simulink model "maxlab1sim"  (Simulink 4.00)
settings: Solver=ode45  SolverMode=SingleTasking  StartTime=0.0  StopTime=2  FixedStep=0.001  RelTol=1e-3
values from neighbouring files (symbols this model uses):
  C = lC    [initlab1sim.m]
  dDZ = 0.1    [initlab1sim.m]
  dzpos = 0    [initlab1sim.m]
  DZPOS = 0    [initlab1sim.m]
  GAM = lGAM    [initlab1sim.m]
  h = 0.001    [dfa.m]    (also in initlab1sim.m)
  K = lK    [initlab1sim.m]    (also in lqed.m = Phi*Kf+Kv)
  Lc = lLc    (= 1)    [initlab1sim.m]
  Le = lLe    [initlab1sim.m]
  overlap = 0    [fix_opencfg.m]    (also in fixopencfg.m; initlab1sim.m)
  OVERLAP = 2    [initlab1sim.m]
  PHI = lPHI    [initlab1sim.m]
  tl = -1.3    [initlab1sim.m]
  TL = + 1.3    (= 1.3)    [initlab1sim.m]
  tu = 1.0    (= 1)    [initlab1sim.m]
  TU = - 1.0    (= -1)    [initlab1sim.m]
undefined symbols (not defined in the file or in its folder): SimDen, SimNum
libraries: simulink3 x2, simulink_extras x1

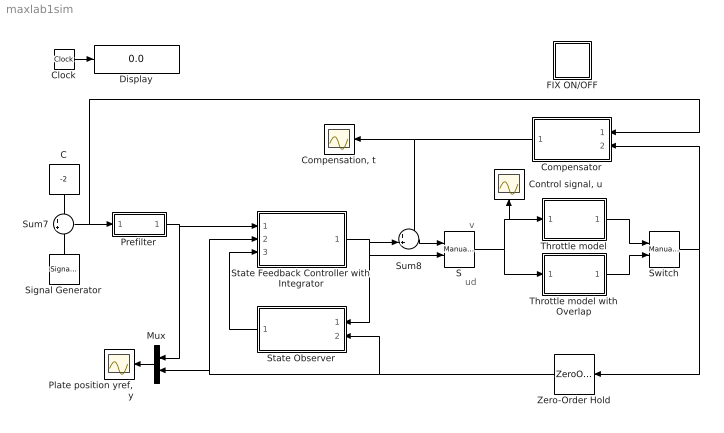
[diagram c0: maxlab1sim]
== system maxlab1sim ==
  note: v
  note: ud
  C : Constant  Orientation=down  Value=-2
  Clock : Clock
  "Compensation, t" : Scope
  Compensator : Subsystem  Orientation=left
  "Control signal, u" : Scope
  Display : Display
  FIX ON/OFF : Subsystem  Description=Fix ON/OFF
  Mux : Mux  Orientation=left  Inputs=2
  "Plate position yref, y" : Scope
  Prefilter : Subsystem
  S : simulink3/Nonlinear/Manual Switch  sw=0  action=0
  Signal Generator : SignalGenerator  Orientation=up  WaveForm=square  Amplitude=2  Frequency=1  Units=Hertz
  State Feedback Controller with Integrator : Subsystem
  State Observer : Subsystem  Orientation=left
  Sum7 : Sum  Inputs=++  SaturateOnIntegerOverflow=on
  Sum8 : Sum  Inputs=++|  SaturateOnIntegerOverflow=on
  Switch : simulink3/Nonlinear/Manual Switch  sw=1  action=0
  Throttle model : Subsystem
  Throttle model with Overlap : Subsystem
  Zero-Order Hold : ZeroOrderHold  Orientation=left  SampleTime=h
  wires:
  Signal Generator/1 -> Sum7/2
  Prefilter/1(rfiltered) -> Mux/1, State Feedback Controller with Integrator/1(yr)
  Mux/1 -> "Plate position yref, y"/1
  Zero-Order Hold/1 -> State Observer/2(y), Mux/2, State Feedback Controller with Integrator/2(y)
  State Observer/1(xhat) -> State Feedback Controller with Integrator/3(xhat)
  Sum7/1 -> Prefilter/1(r), Compensator/1(ref.value)
  Switch/1 -> Zero-Order Hold/1, Compensator/2(y)
  Sum8/1 -> S/1
  State Feedback Controller with Integrator/1(ud) -> Sum8/2, S/2, State Observer/1(u)
  Throttle model with Overlap/1(y) -> Switch/2
  Throttle model/1(y) -> Switch/1
  S/1 -> Throttle model/1(u), "Control signal, u"/1, Throttle model with Overlap/1(u)
  Compensator/1(t) -> Sum8/1, "Compensation, t"/1
  Clock/1 -> Display/1
  C/1 -> Sum7/1

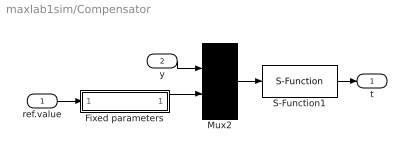
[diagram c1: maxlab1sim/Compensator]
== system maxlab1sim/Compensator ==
  ref.value : Inport  Port=1  LatchInput=off
  y : Inport  Port=2  LatchInput=off
  Fixed parameters : Subsystem
  Mux2 : Mux  Inputs=2
  S-Function1 : S-Function  FunctionName=compensator2  Parameters=h overlap/2 -overlap/2  PortCounts=[]  SFunctionModules=''
  t : Outport  Port=1
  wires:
  ref.value/1 -> Fixed parameters/1(ref value)
  y/1 -> Mux2/1
  Mux2/1 -> S-Function1/1
  S-Function1/1 -> t/1
  Fixed parameters/1(params) -> Mux2/2

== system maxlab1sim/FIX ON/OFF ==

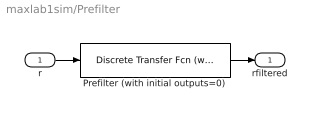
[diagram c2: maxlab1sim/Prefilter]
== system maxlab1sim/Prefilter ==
  r : Inport  Port=1  LatchInput=off
  Prefilter (with initial outputs=0) : simulink_extras/Additional Discrete/Discrete Transfer Fcn (with initial outputs)  N=[21.3 1 -20.3]  D=[835 -1596 763]  U0=[0]  Y0=0  TS=h
  rfiltered : Outport  Port=1
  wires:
  Prefilter (with initial outputs=0)/1 -> rfiltered/1
  r/1 -> Prefilter (with initial outputs=0)/1

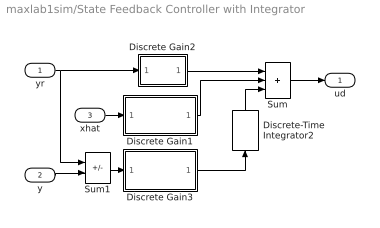
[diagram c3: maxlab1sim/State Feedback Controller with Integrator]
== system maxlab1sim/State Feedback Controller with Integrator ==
  yr : Inport  Port=1  LatchInput=off
  y : Inport  Port=2  LatchInput=off
  xhat : Inport  Port=3  LatchInput=off
  Discrete Gain1 : Subsystem  mask(Discrete Gain){h=h, K=-Le(1:3)}
      mask prompts: h "Sample Time"; K "Gain"
      mask init:
      | s = get_param(gcb,'MaskValueString');
      | s = s(findstr(s,'|')+1:end);
  Discrete Gain2 : Subsystem  mask(Discrete Gain){h=h, K=Lc}
      mask prompts: h "Sample Time"; K "Gain"
      mask init:
      | s = get_param(gcb,'MaskValueString');
      | s = s(findstr(s,'|')+1:end);
  Discrete Gain3 : Subsystem  mask(Discrete Gain){h=h, K=-Le(4)}
      mask prompts: h "Sample Time"; K "Gain"
      mask init:
      | s = get_param(gcb,'MaskValueString');
      | s = s(findstr(s,'|')+1:end);
  Discrete-Time Integrator2 : DiscreteIntegrator  Orientation=up  IntegratorMethod=ForwardEuler  ExternalReset=none  InitialConditionSource=internal  InitialCondition=0  LimitOutput=off  UpperSaturationLimit=inf  LowerSaturationLimit=-inf  ShowSaturationPort=off  ShowStatePort=off  SampleTime=h
  Sum : Sum  Inputs=+++  SaturateOnIntegerOverflow=on
  Sum1 : Sum  Inputs=+-  SaturateOnIntegerOverflow=on
  ud : Outport  Port=1
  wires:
  Discrete Gain1/1(Out1) -> Sum/2
  Discrete-Time Integrator2/1 -> Sum/3
  Sum/1 -> ud/1
  Discrete Gain3/1(Out1) -> Discrete-Time Integrator2/1
  Discrete Gain2/1(Out1) -> Sum/1
  xhat/1 -> Discrete Gain1/1(In1)
  y/1 -> Sum1/2
  yr/1 -> Discrete Gain2/1(In1), Sum1/1
  Sum1/1 -> Discrete Gain3/1(In1)

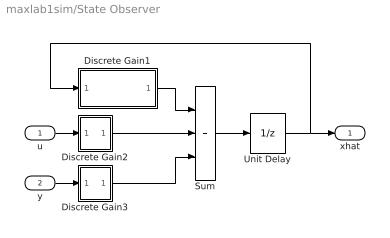
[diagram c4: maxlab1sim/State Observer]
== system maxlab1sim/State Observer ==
  u : Inport  Port=1  LatchInput=off
  y : Inport  Port=2  LatchInput=off
  Discrete Gain1 : Subsystem  mask(Discrete Gain){h=h, K=PHI-K*C}
      mask prompts: h "Sample Time"; K "Gain"
      mask init:
      | s = get_param(gcb,'MaskValueString');
      | s = s(findstr(s,'|')+1:end);
  Discrete Gain2 : Subsystem  mask(Discrete Gain){h=h, K=GAM}
      mask prompts: h "Sample Time"; K "Gain"
      mask init:
      | s = get_param(gcb,'MaskValueString');
      | s = s(findstr(s,'|')+1:end);
  Discrete Gain3 : Subsystem  mask(Discrete Gain){h=h, K=K}
      mask prompts: h "Sample Time"; K "Gain"
      mask init:
      | s = get_param(gcb,'MaskValueString');
      | s = s(findstr(s,'|')+1:end);
  Sum : Sum  Inputs=+++  SaturateOnIntegerOverflow=on
  Unit Delay : UnitDelay  X0=0  SampleTime=h
  xhat : Outport  Port=1
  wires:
  Discrete Gain1/1(Out1) -> Sum/1
  Discrete Gain2/1(Out1) -> Sum/2
  Discrete Gain3/1(Out1) -> Sum/3
  Sum/1 -> Unit Delay/1
  Unit Delay/1 -> Discrete Gain1/1(In1), xhat/1
  u/1 -> Discrete Gain2/1(In1)
  y/1 -> Discrete Gain3/1(In1)

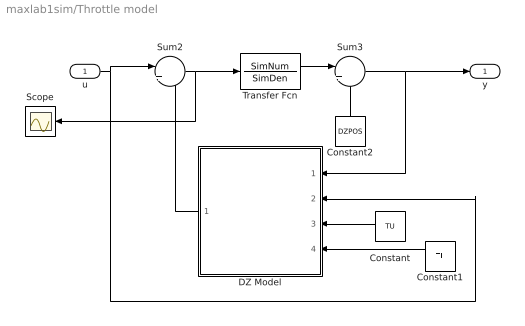
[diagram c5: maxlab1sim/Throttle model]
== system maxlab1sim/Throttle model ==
  u : Inport  Port=1  LatchInput=off
  Constant : Constant  Orientation=left  Value=TU
  Constant1 : Constant  Orientation=left  Value=TL
  Constant2 : Constant  Orientation=up  Value=DZPOS
  DZ Model : Subsystem  Orientation=left
  Scope : Scope
  Sum2 : Sum  Inputs=|++  SaturateOnIntegerOverflow=on
  Sum3 : Sum  Inputs=|++  SaturateOnIntegerOverflow=on
  Transfer Fcn : TransferFcn  Numerator=SimNum  Denominator=SimDen  AbsoluteTolerance=auto  Realization=auto
  y : Outport  Port=1
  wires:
  Sum3/1 -> DZ Model/1(position), y/1
  Constant2/1 -> Sum3/2
  Transfer Fcn/1 -> Sum3/1
  u/1 -> DZ Model/2(torque), Sum2/1
  Constant/1 -> DZ Model/3(TU)
  Constant1/1 -> DZ Model/4(TL)
  Sum2/1 -> Transfer Fcn/1, Scope/1
  DZ Model/1(dz) -> Sum2/2

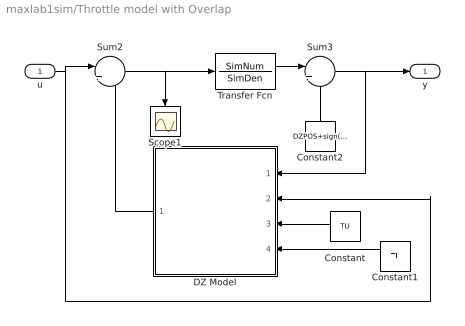
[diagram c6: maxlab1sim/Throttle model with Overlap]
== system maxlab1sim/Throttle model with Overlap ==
  u : Inport  Port=1  LatchInput=off
  Constant : Constant  Orientation=left  Value=TU
  Constant1 : Constant  Orientation=left  Value=TL
  Constant2 : Constant  Orientation=up  Value=DZPOS+sign(TU+TL)*OVERLAP/2
  DZ Model : Subsystem  Orientation=left
  Scope1 : Scope
  Sum2 : Sum  Inputs=|++  SaturateOnIntegerOverflow=on
  Sum3 : Sum  Inputs=|++  SaturateOnIntegerOverflow=on
  Transfer Fcn : TransferFcn  Numerator=SimNum  Denominator=SimDen  AbsoluteTolerance=auto  Realization=auto
  y : Outport  Port=1
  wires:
  Sum3/1 -> DZ Model/1(position), y/1
  Constant2/1 -> Sum3/2
  Transfer Fcn/1 -> Sum3/1
  Sum2/1 -> Scope1/1, Transfer Fcn/1
  Constant1/1 -> DZ Model/4(TL)
  Constant/1 -> DZ Model/3(TU)
  u/1 -> DZ Model/2(torque), Sum2/1
  DZ Model/1(dz) -> Sum2/2

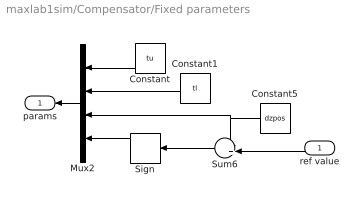
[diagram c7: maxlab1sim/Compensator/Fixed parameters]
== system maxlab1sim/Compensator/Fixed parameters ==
  ref value : Inport  Orientation=left  Port=1  LatchInput=off
  Constant : Constant  Orientation=left  Value=tu
  Constant1 : Constant  Orientation=left  Value=tl
  Constant5 : Constant  Orientation=left  Value=dzpos
  Mux2 : Mux  Orientation=left  Inputs=4
  Sign : Signum  Orientation=left
  Sum6 : Sum  Orientation=left  Inputs=-+|  SaturateOnIntegerOverflow=on
  params : Outport  Orientation=left  Port=1
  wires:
  Sign/1 -> Mux2/4
  Constant/1 -> Mux2/1
  Constant5/1 -> Mux2/3, Sum6/1
  ref value/1 -> Sum6/2
  Sum6/1 -> Sign/1
  Constant1/1 -> Mux2/2
  Mux2/1 -> params/1

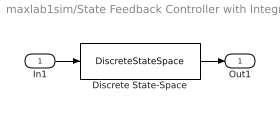
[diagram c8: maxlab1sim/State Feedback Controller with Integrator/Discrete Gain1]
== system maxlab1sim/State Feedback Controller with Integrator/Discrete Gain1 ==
  In1 : Inport  Port=1  LatchInput=off
  Discrete State-Space : DiscreteStateSpace  A=0  B=zeros(1,size(K,2))  C=zeros(size(K,1),1)  D=K  X0=0  SampleTime=h  Realization=auto
  Out1 : Outport  Port=1
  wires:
  Discrete State-Space/1 -> Out1/1
  In1/1 -> Discrete State-Space/1

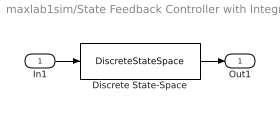
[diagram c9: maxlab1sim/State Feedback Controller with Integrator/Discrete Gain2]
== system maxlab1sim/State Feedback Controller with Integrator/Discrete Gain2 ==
  In1 : Inport  Port=1  LatchInput=off
  Discrete State-Space : DiscreteStateSpace  A=0  B=zeros(1,size(K,2))  C=zeros(size(K,1),1)  D=K  X0=0  SampleTime=h  Realization=auto
  Out1 : Outport  Port=1
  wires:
  Discrete State-Space/1 -> Out1/1
  In1/1 -> Discrete State-Space/1

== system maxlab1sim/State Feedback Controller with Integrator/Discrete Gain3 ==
  In1 : Inport  Port=1  LatchInput=off
  Discrete State-Space : DiscreteStateSpace  A=0  B=zeros(1,size(K,2))  C=zeros(size(K,1),1)  D=K  X0=0  SampleTime=h  Realization=auto
  Out1 : Outport  Port=1
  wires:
  In1/1 -> Discrete State-Space/1
  Discrete State-Space/1 -> Out1/1

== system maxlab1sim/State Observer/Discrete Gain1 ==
  In1 : Inport  Port=1  LatchInput=off
  Discrete State-Space : DiscreteStateSpace  A=0  B=zeros(1,size(K,2))  C=zeros(size(K,1),1)  D=K  X0=0  SampleTime=h  Realization=auto
  Out1 : Outport  Port=1
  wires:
  Discrete State-Space/1 -> Out1/1
  In1/1 -> Discrete State-Space/1

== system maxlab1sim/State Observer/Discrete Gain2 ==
  In1 : Inport  Port=1  LatchInput=off
  Discrete State-Space : DiscreteStateSpace  A=0  B=zeros(1,size(K,2))  C=zeros(size(K,1),1)  D=K  X0=0  SampleTime=h  Realization=auto
  Out1 : Outport  Port=1
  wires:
  In1/1 -> Discrete State-Space/1
  Discrete State-Space/1 -> Out1/1

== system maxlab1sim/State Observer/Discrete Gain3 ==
  In1 : Inport  Port=1  LatchInput=off
  Discrete State-Space : DiscreteStateSpace  A=0  B=zeros(1,size(K,2))  C=zeros(size(K,1),1)  D=K  X0=0  SampleTime=h  Realization=auto
  Out1 : Outport  Port=1
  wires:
  Discrete State-Space/1 -> Out1/1
  In1/1 -> Discrete State-Space/1

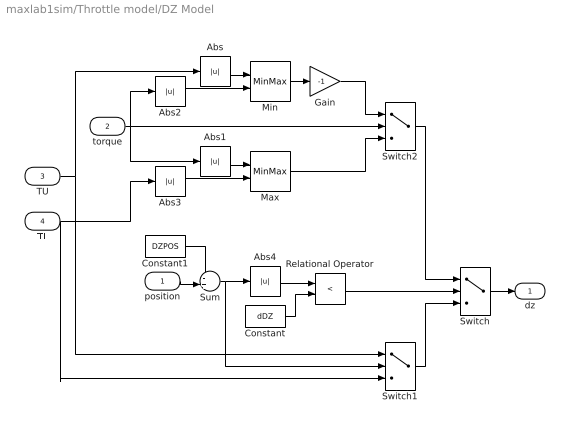
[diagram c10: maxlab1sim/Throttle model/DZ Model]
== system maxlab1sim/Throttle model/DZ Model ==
  position : Inport  Port=1  LatchInput=off
  torque : Inport  Port=2  LatchInput=off
  TU : Inport  Port=3  LatchInput=off
  TL : Inport  Port=4  LatchInput=off
  Abs{,1..4} (5 alike) : Abs  SaturateOnIntegerOverflow=on
  Constant : Constant  Value=dDZ
  Constant1 : Constant  Value=DZPOS
  Gain : Gain  Gain=-1  Multiplication=Element-wise(K.*u)  SaturateOnIntegerOverflow=on
  Max : MinMax  Function=min  Inputs=2
  Min : MinMax  Function=min  Inputs=2
  Relational Operator : RelationalOperator  Operator=<
  Sum : Sum  Inputs=-+|  SaturateOnIntegerOverflow=on
  Switch : Switch  Threshold=0.5
  Switch1 : Switch  Threshold=0
  Switch2 : Switch  Threshold=0
  dz : Outport  Port=1  InitialOutput=0
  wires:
  Abs4/1 -> Relational Operator/1
  Relational Operator/1 -> Switch/2
  Max/1 -> Switch2/3
  TL/1 -> Switch1/3, Abs3/1
  torque/1 -> Switch2/2, Abs1/1, Abs2/1
  TU/1 -> Switch1/1, Abs/1
  Abs/1 -> Min/1
  Abs1/1 -> Max/1
  Min/1 -> Gain/1
  Gain/1 -> Switch2/1
  Abs2/1 -> Min/2
  Abs3/1 -> Max/2
  Switch2/1 -> Switch/1
  Switch1/1 -> Switch/3
  Switch/1 -> dz/1
  Constant/1 -> Relational Operator/2
  position/1 -> Sum/2
  Constant1/1 -> Sum/1
  Sum/1 -> Abs4/1, Switch1/2

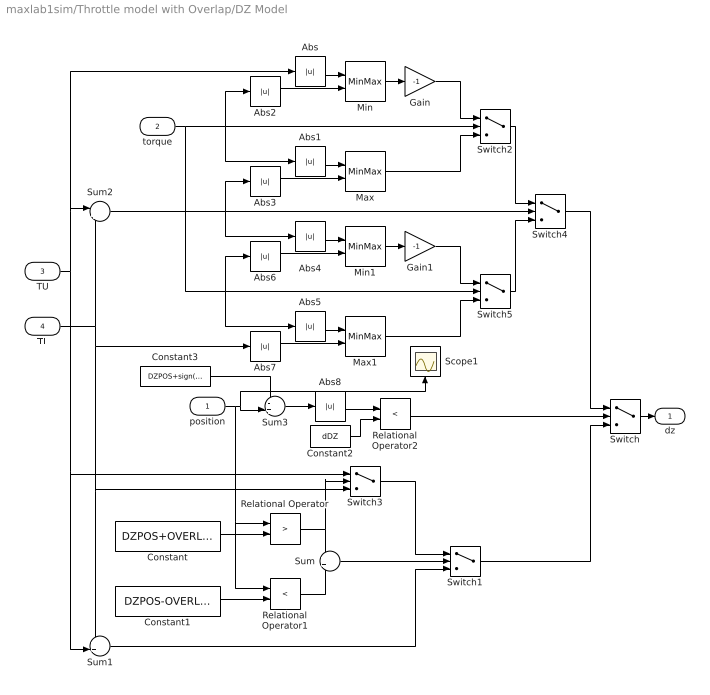
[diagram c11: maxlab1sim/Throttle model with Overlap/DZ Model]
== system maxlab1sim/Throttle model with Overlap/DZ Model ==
  position : Inport  Port=1  LatchInput=off
  torque : Inport  Port=2  LatchInput=off
  TU : Inport  Port=3  LatchInput=off
  TL : Inport  Port=4  LatchInput=off
  Abs{,1..8} (9 alike) : Abs  SaturateOnIntegerOverflow=on
  Constant : Constant  Value=DZPOS+OVERLAP/2
  Constant1 : Constant  Value=DZPOS-OVERLAP/2
  Constant2 : Constant  Value=dDZ
  Constant3 : Constant  Value=DZPOS+sign(TU+TL)*OVERLAP/2
  Gain : Gain  Gain=-1  Multiplication=Element-wise(K.*u)  SaturateOnIntegerOverflow=on
  Gain1 : Gain  Gain=-1  Multiplication=Element-wise(K.*u)  SaturateOnIntegerOverflow=on
  Max : MinMax  Function=min  Inputs=2
  Max1 : MinMax  Function=min  Inputs=2
  Min : MinMax  Function=min  Inputs=2
  Min1 : MinMax  Function=min  Inputs=2
  Relational Operator : RelationalOperator  Operator=>
  Relational Operator1 : RelationalOperator  Operator=<
  Relational Operator2 : RelationalOperator  Operator=<
  Scope1 : Scope
  Sum : Sum  Inputs=++  SaturateOnIntegerOverflow=on
  Sum1 : Sum  Inputs=++|  SaturateOnIntegerOverflow=on
  Sum2 : Sum  Inputs=|++  SaturateOnIntegerOverflow=on
  Sum3 : Sum  Inputs=-+|  SaturateOnIntegerOverflow=on
  Switch : Switch  Threshold=0.5
  Switch1 : Switch  Threshold=0.5
  Switch2 : Switch  Threshold=0
  Switch3 : Switch  Threshold=0.5
  Switch4 : Switch  Threshold=0
  Switch5 : Switch  Threshold=0
  dz : Outport  Port=1  InitialOutput=0
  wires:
  Abs8/1 -> Relational Operator2/1
  Relational Operator2/1 -> Switch/2
  Sum3/1 -> Abs8/1
  Constant2/1 -> Relational Operator2/2
  Constant3/1 -> Sum3/1
  position/1 -> Scope1/1, Sum3/2, Relational Operator/1, Relational Operator1/1
  TL/1 -> Sum2/2, Sum1/1, Switch3/3, Abs7/1
  TU/1 -> Switch3/1, Sum1/2, Sum2/1, Abs/1
  Abs/1 -> Min/1
  Abs1/1 -> Max/1
  Min/1 -> Gain/1
  Gain/1 -> Switch2/1
  Abs2/1 -> Min/2
  Abs3/1 -> Max/2
  Max1/1 -> Switch5/3
  Abs4/1 -> Min1/1
  Abs5/1 -> Max1/1
  Abs6/1 -> Min1/2
  Abs7/1 -> Max1/2
  Constant/1 -> Relational Operator/2
  Constant1/1 -> Relational Operator1/2
  Relational Operator1/1 -> Sum/2
  Sum/1 -> Switch1/2
  Sum1/1 -> Switch1/3
  Switch3/1 -> Switch1/1
  Relational Operator/1 -> Sum/1, Switch3/2
  Switch1/1 -> Switch/3
  torque/1 -> Switch2/2, Abs1/1, Abs2/1, Switch5/2, Abs6/1, Abs5/1
  Switch2/1 -> Switch4/1
  Switch5/1 -> Switch4/3
  Switch/1 -> dz/1
  Switch4/1 -> Switch/1
  Sum2/1 -> Switch4/2, Abs3/1, Abs4/1
  Max/1 -> Switch2/3
  Min1/1 -> Gain1/1
  Gain1/1 -> Switch5/1
